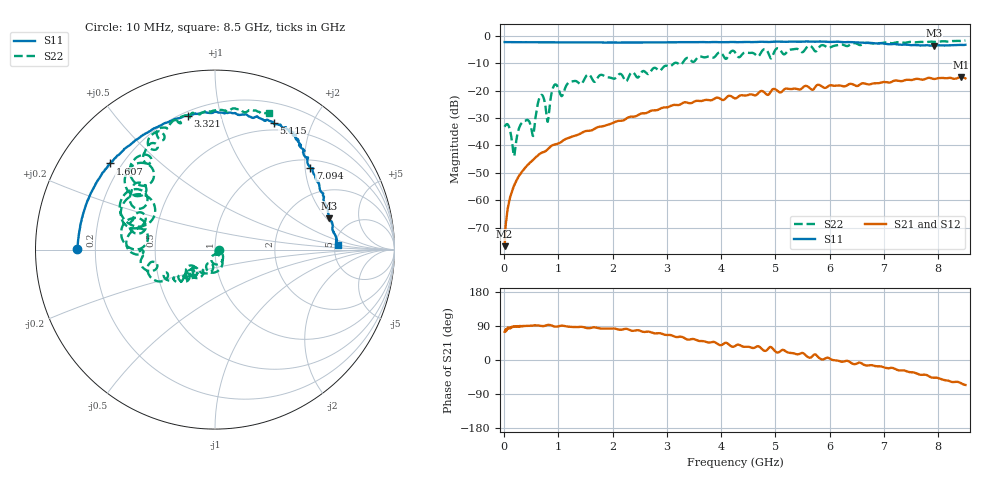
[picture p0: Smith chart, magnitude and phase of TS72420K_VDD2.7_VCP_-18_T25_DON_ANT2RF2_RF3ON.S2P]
!Agilent Technologies,E5071C,MY46417908,A.11.23
!Date: Thu Oct 03 16:41:21 2019
!Data & Calibration Information:
!Freq	S11:SOLT2(ON)	S21:SOLT2(ON)	S12:SOLT2(ON)	S22:SOLT2(ON)
!PortZ  Port1:50+j0  Port2:50+j0
!Above PortZ is port z conversion or system Z0 setting when saving the data.
!When reading, reference impedance value at option line is always used.
# Hz S dB R 50
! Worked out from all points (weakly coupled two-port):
!   1601 points, 10 MHz to 8.5 GHz, reference 50 ohm
!   highest |S21| = -15.03 dB at 8.42 GHz (marker M1); lowest = -76.8 dB at 10 MHz (marker M2)
!   lowest |S11| = -3.6 dB at 7.922 GHz (marker M3), VSWR 4.85, Z = 173 + j106 ohm
!   |S11| at or under -10 dB: nowhere
!   |S22| runs from -43.9 to -1.7 dB; largest |S21 - S12| = 0.002
!   S11 on the Smith chart (normalised r, x): 10 MHz: 0.13, +0.00; 1.607 GHz: 0.16, +0.35; 3.321 GHz: 0.22, +0.79; 5.115 GHz: 0.42, +1.48; 7.094 GHz: 1.19, +2.13; 8.5 GHz: 5.28, +0.55
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1e7  -2.29 179.8  -76.76 74.7  -76.84 68.7  -33.19 -0.3
8.42875e7  -2.32 177.7  -61.48 83.1  -61.36 82.6  -32.87 -38.9
1.851062e8  -2.34 175.1  -54.69 88.4  -54.74 87.4  -43.86 -36.8
3.28375e8  -2.35 171.3  -49.64 89.4  -49.67 89.2  -31.77 -44.0
5.353188e8  -2.37 166.0  -45.27 90.8  -45.30 91.0  -36.59 -52.0
6.838938e8  -2.38 162.3  -42.75 89.8  -42.80 89.8  -21.59 -76.4
8.059375e8  -2.37 159.4  -41.39 92.6  -41.43 92.3  -31.37 -80.0
9.385938e8  -2.39 156.0  -39.64 88.3  -39.66 88.1  -17.78 -94.2
1.060638e9  -2.40 153.3  -38.62 90.7  -38.63 90.4  -22.03 -108.5
1.203906e9  -2.40 149.8  -37.16 87.6  -37.18 87.5  -16.95 -110.6
1.426769e9  -2.42 144.8  -35.49 87.4  -35.49 87.2  -17.55 -121.1
1.607181e9  -2.43 140.6  -34.56 84.9  -34.55 84.7  -15.16 -140.3
2.843538e9  -2.41 111.7  -26.96 70.8  -26.91 70.8  -12.61 -143.7
3.3211e9  -2.36 101.5  -24.31 58.1  -24.27 58.2  -8.97 -150.0
4.255e9  -2.29 81.4  -22.85 36.8  -22.84 37.0  -6.02 159.9
5.114612e9  -2.20 65.1  -20.45 25.9  -20.44 26.0  -5.94 140.9
5.671769e9  -2.16 57.7  -19.69 8.7  -19.67 8.8  -4.12 129.2
7.088538e9  -3.10 41.0  -17.08 -21.8  -17.12 -21.7  -2.54 105.8
7.093844e9  -3.11 40.7  -17.09 -21.7  -17.12 -21.6  -2.56 105.6
7.921619e9  -3.64 15.3  -15.77 -46.6  -15.67 -46.6  -2.20 85.8
8.420406e9  -3.33 4.3  -15.03 -61.4  -15.04 -61.5  -1.88 71.1
8.5e9  -3.29 2.3  -15.56 -65.8  -15.63 -65.9  -1.72 68.5
